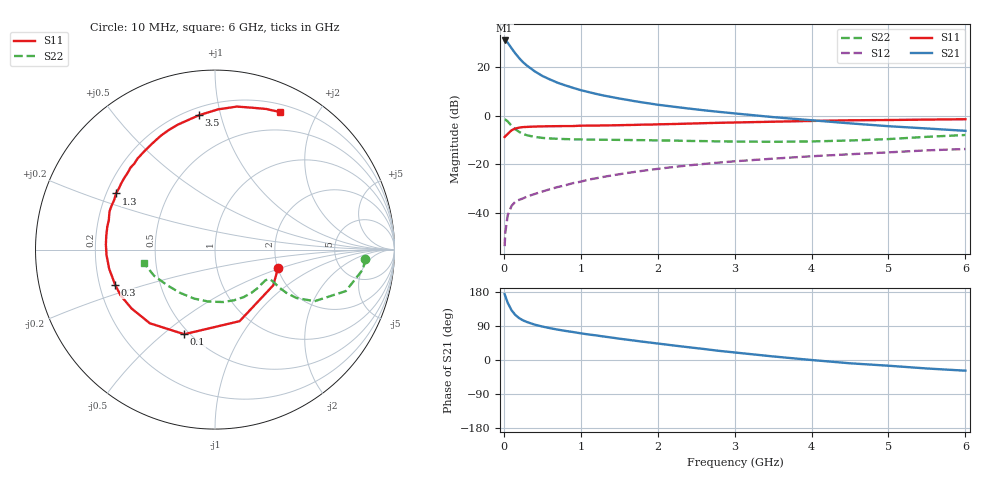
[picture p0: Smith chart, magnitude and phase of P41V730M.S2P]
! SIEMENS Small Signal Semiconductors
! BFP182
! Si NPN RF Bipolar Junction Transistor in SOT143
! VCE = 1.75 V  IC = 30 mA
! Common Emitter S-Parameters:  March  1996
# GHz  S  MA  R  50
!  f  S11  S21  S12  S22
! GHz  MAG  ANG  MAG  ANG  MAG  ANG  MAG  ANG
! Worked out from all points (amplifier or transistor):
!   36 points, 10 MHz to 6 GHz, reference 50 ohm
!   highest |S21| = 30.9 dB at 10 MHz (marker M1)
!   |S21| within 3 dB of that: start of sweep to 95.91 MHz
!   unconditionally stable (mu >= 1): start of sweep to 18.61 MHz; 263.7 MHz to end of sweep
!   at 250 MHz: K = 0.97, MSG = 27.9 dB, |S12| = -33.9 dB
!   at 1.4 GHz: K = 1.73, MAG = 11.1 dB, |S12| = -24.5 dB
!   at 6 GHz: K = 1.23, MAG = 0.9 dB, |S12| = -13.7 dB
!   S11 on the Smith chart (normalised r, x): 10 MHz: 2.01, -0.48; 100 MHz: 0.47, -0.59; 300 MHz: 0.27, -0.16; 1.3 GHz: 0.24, +0.25; 3.5 GHz: 0.25, +0.86; 6 GHz: 0.28, +1.54
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0.01  0.3656 -16.3  35.1 173.9  0.0021 79.4  0.8393 -3.5
0.02  0.3809 -31.4  34.83 168.1  0.0041 73.7  0.8317 -7.6
0.05  0.4217 -71.0  31.62 151.2  0.009 69.5  0.7645 -17.6
0.1  0.5018 -110.0  24.32 131.3  0.0141 52.2  0.6249 -27.4
0.15  0.548 -131.5  18.96 118.8  0.0172 47.5  0.5281 -30.7
0.2  0.5692 -144.9  15.18 110.4  0.0188 45.7  0.4639 -31.2
0.25  0.5847 -154.1  12.53 104.5  0.0201 46.2  0.4239 -30.7
0.3  0.5898 -160.5  10.7 100.3  0.0219 46.5  0.3971 -29.9
0.4  0.5993 -169.7  8.192 93.3  0.0247 48.9  0.3676 -28.8
0.5  0.6052 -177.1  6.568 88.3  0.0278 50.8  0.3507 -28.5
0.6  0.6087 177.2  5.552 84.0  0.031 52.9  0.3416 -28.8
0.7  0.6108 172.6  4.748 80.2  0.0344 54.4  0.3357 -29.6
0.8  0.6136 167.9  4.198 76.8  0.0373 55.9  0.3317 -30.7
1.1  0.6261 157.0  3.066 67.4  0.0487 56.9  0.3241 -35.2
1.3  0.634 150.4  2.593 61.9  0.0557 57.0  0.3211 -38.8
1.7  0.6485 138.3  1.99 51.1  0.0702 55.7  0.316 -47.1
2.2  0.6755 125.3  1.537 38.5  0.0883 52.4  0.3093 -58.9
2.8  0.7156 110.7  1.199 24.1  0.1093 47.1  0.2969 -75.3
3.5  0.7537 96.9  0.937 9.4  0.1315 40.6  0.2918 -97.0
4.5  0.8061 81.3  0.697 -8.7  0.1619 31.3  0.31 -129.2
5.5  0.8337 70.0  0.547 -22.4  0.1947 22.0  0.3691 -156.7
6  0.8472 64.8  0.49 -28.2  0.2073 16.3  0.4026 -169.0
